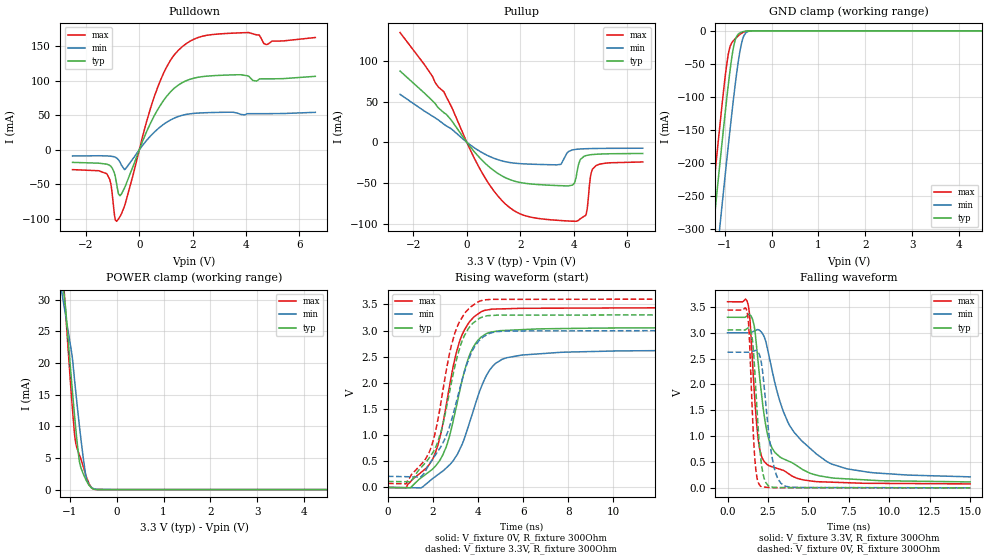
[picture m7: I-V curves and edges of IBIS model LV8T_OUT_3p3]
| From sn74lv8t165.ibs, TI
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[Model]   LV8T_OUT_3p3
Model_type   3-state
Polarity   Non-Inverting
Vmeas = 1.65
Vref = 0
Cref = 50pF
Rref = 1000
|   typ   min   max
C_comp   1.25pF   1.25pF   1.25pF
[Voltage Range]   3.3   3   3.6
[Temperature Range]   27   125   -40
[Pullup Reference]   3.3   3   3.6
[Pulldown Reference]   0   0   0
[Power Clamp Reference]   3.3   3   3.6
[GND Clamp Reference]   0   0   0
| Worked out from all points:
|   slope of the pulldown table from 0 to 0.495 V, typ, clamps not added: 11.2 ohm
|   slope of the pullup table from 0 to 0.495 V, typ, clamps not added: 25.4 ohm
|   GND clamp passes 1 mA (typ) near -0.60 V on its own axis
|   POWER clamp passes 1 mA (typ) near -0.62 V on its own axis
|   falling waveform, V_fixture 3.3V, R_fixture 300Ohm: 20-80 % time 967ps typ, 2.44ns min, 513ps max; typ from 3.3 V to 0.115 V
|   rising waveform, V_fixture 0V, R_fixture 300Ohm: 20-80 % time 1.13ns typ, 1.41ns min, 1.03ns max; typ from 0 V to 3.05 V
|   rising waveform, V_fixture 3.3V, R_fixture 300Ohm: 20-80 % time 1.09ns typ, 1.24ns min, 1.01ns max; typ from 0.115 V to 3.3 V
|   falling waveform, V_fixture 0V, R_fixture 300Ohm: 20-80 % time 392ps typ, 575ps min, 290ps max; typ from 3.05 V to 0 V
[Pulldown]
|   Voltage   I(typ)   I(min)   I(max)
-2.5V     -18.28mA   -9.059mA   -28.76mA
-1.219V   -20.85mA   -8.945mA   -34.73mA
-1.072V   -23.75mA   -9.364mA   -48.57mA
-851.5mV  -49.06mA   -11.94mA   -103.5mA
-673mV    -64.24mA   -22.03mA   -92.85mA
-526mV    -52.66mA   -28.15mA   -77.89mA
576.5mV   50.36mA    25.98mA    78.49mA
1.458V    93.46mA    48.05mA    143.7mA
2.781V    107.1mA    53.86mA    166.7mA
4.104V    106.1mA    52.14mA    169.4mA
4.766V    102.5mA    52.18mA    152mA
6.593V    106.1mA    54.08mA    162.3mA
[GND Clamp]
|   Voltage   I(typ)   I(min)   I(max)
-2.5V     -1.223A    -1.308A    -1.175A
-1.313V   -348.7mA   -443.1mA   -291.5mA
-1.23V    -288.7mA   -383.5mA   -231.1mA
-1.135V   -222.2mA   -317.2mA   -164.4mA
-1.062V   -171.5mA   -266.3mA   -114.2mA
-977.5mV  -115.5mA   -209.1mA   -61.53mA
-904mV    -69.7mA    -160.4mA   -28.36mA
-778mV    -14.25mA   -82.1mA    -12.14mA
-631mV    -1.745mA   -15.92mA   -3.28mA
-547mV    -376.1uA   -2.828mA   -696.1uA
-431.5mV  -13.18uA   -139.1uA   -11.29uA
8V        0A         0A         0A
[Pullup]
|   Voltage   I(typ)   I(min)   I(max)
-2.5V     87.68mA    59.03mA    135.1mA
-862mV    36.51mA    22.33mA    62.28mA
818mV     -29.69mA   -16.88mA   -50.68mA
1.899V    -48.81mA   -26.05mA   -86.57mA
3.517V    -53.44mA   -27.19mA   -96.33mA
3.968V    -52.42mA   -9.344mA   -97.17mA
4.115V    -39.24mA   -8.613mA   -97.14mA
4.252V    -21.24mA   -8.244mA   -94.22mA
4.472V    -16.35mA   -7.907mA   -88.73mA
4.64V     -15.34mA   -7.753mA   -41.15mA
4.84V     -14.75mA   -7.63mA    -28.74mA
6.593V    -13.76mA   -7.306mA   -24.22mA
[POWER Clamp]
|   Voltage   I(typ)   I(min)   I(max)
-2.5V     124.4mA    98.39mA    156.4mA
-1.177V   34.15mA    31.45mA    37.71mA
-1.093V   28.93mA    27.63mA    28.34mA
-956.5mV  16.59mA    21.43mA    13.96mA
-904mV    12.13mA    17.74mA    9.183mA
-883mV    10.43mA    16.19mA    7.781mA
-830.5mV  6.564mA    12.45mA    6.182mA
-788.5mV  4.183mA    9.635mA    5.343mA
-662.5mV  1.647mA    2.362mA    2.407mA
-589mV    682.9uA    753.1uA    922.8uA
-494.5mV  92.62uA    157.9uA    70.62uA
8V        0A         0A         0A
[Ramp]
R_load = 300
|   typ   min   max
dV/dt_r   1.83253/1.12668e-09   1.57402/1.40448e-09   2.06332/1.02106e-09
dV/dt_f   1.91099/9.65039e-10   1.6721/2.43384e-09   2.11391/5.13e-10
[Falling Waveform]
V_fixture = 3.3V
V_fixture_min = 3V
V_fixture_max = 3.6V
R_fixture = 300Ohm
C_fixture = 0F
|   Time   V(typ)   V(min)   V(max)
0s        3.3V       3V         3.6V
1.27ns    3.342V     2.999V     3.552V
1.393ns   3.344V     2.999V     3.227V
1.651ns   3.131V     3.033V     1.884V
1.886ns   2.453V     3.061V     968.4mV
2.457ns   1.056V     2.707V     449.8mV
2.936ns   682.4mV    2.022V     390mV
3.735ns   522.1mV    1.267V     281.9mV
6.108ns   210mV      515.2mV    113.3mV
15ns      114.9mV    212.9mV    76.77mV
[Rising Waveform]
V_fixture = 0V
V_fixture_min = 0V
V_fixture_max = 0V
R_fixture = 300Ohm
C_fixture = 0F
|   Time   V(typ)   V(min)   V(max)
0s        152.2uV    319.6uV    86.61uV
802.1ps   -4.92mV    -4.066mV   -6.019mV
1.692ns   256.2mV    64.39mV    365.6mV
2.327ns   536.6mV    279.5mV    996.6mV
3.159ns   1.792V     703.8mV    2.766V
3.619ns   2.527V     1.237V     3.165V
4.134ns   2.873V     1.913V     3.358V
4.785ns   2.984V     2.375V     3.411V
5.939ns   3.016V     2.531V     3.424V
15ns      3.054V     2.624V     3.439V
[Rising Waveform]
V_fixture = 3.3V
V_fixture_min = 3V
V_fixture_max = 3.6V
R_fixture = 300Ohm
C_fixture = 0F
|   Time   V(typ)   V(min)   V(max)
0s        114.9mV    212.9mV    76.77mV
802.1ps   109.4mV    205.7mV    70.11mV
1.796ns   542.9mV    415.3mV    641.2mV
2.066ns   724.4mV    592.4mV    989.5mV
2.38ns    1.103V     801.7mV    1.701V
2.971ns   2.316V     1.528V     2.954V
3.397ns   2.906V     2.212V     3.323V
3.969ns   3.204V     2.766V     3.541V
4.883ns   3.294V     2.981V     3.596V
15ns      3.3V       3V         3.6V
[Falling Waveform]
|Gnd
V_fixture = 0V
V_fixture_min = 0V
V_fixture_max = 0V
R_fixture = 300Ohm
C_fixture = 0F
|   Time   V(typ)   V(min)   V(max)
0s        3.054V     2.624V     3.439V
1.218ns   3.082V     2.624V     3.392V
1.337ns   3.096V     2.624V     2.987V
1.503ns   2.94V      2.635V     1.703V
1.692ns   2.221V     2.654V     551.8mV
2.066ns   541.7mV    2.461V     26.34mV
2.327ns   129mV      1.758V     13.69mV
2.817ns   10.29mV    484.5mV    4.087mV
3.492ns   4.627mV    44.75mV    3.866mV
15ns      152.2uV    319.6uV    86.59uV
